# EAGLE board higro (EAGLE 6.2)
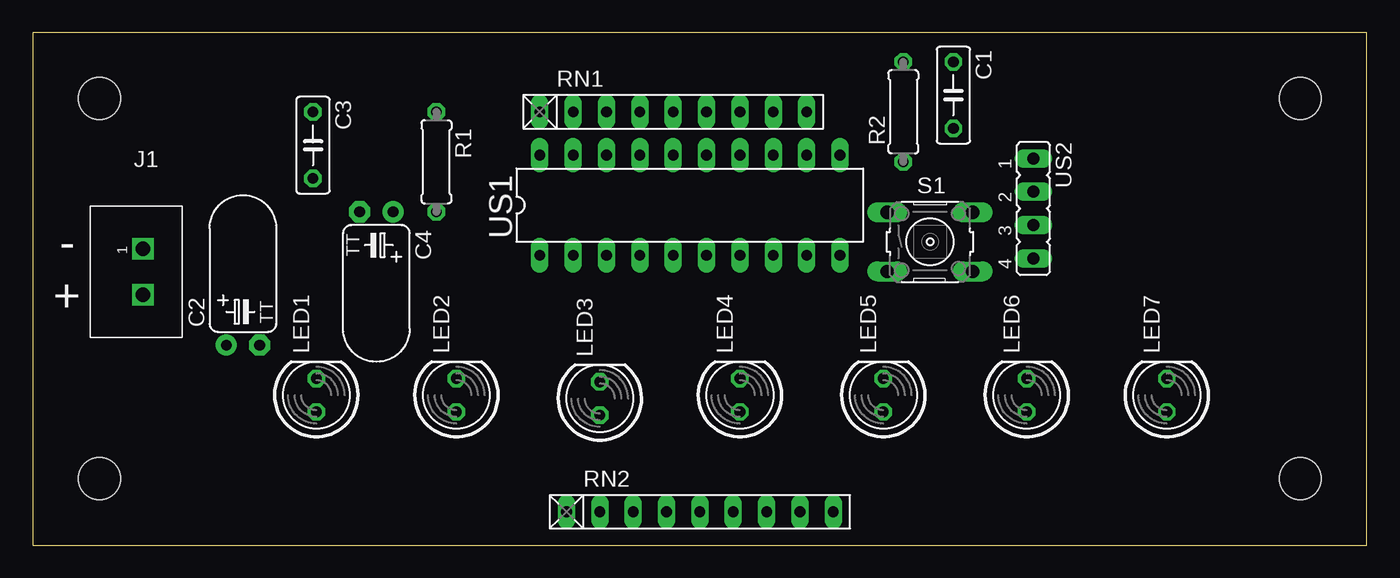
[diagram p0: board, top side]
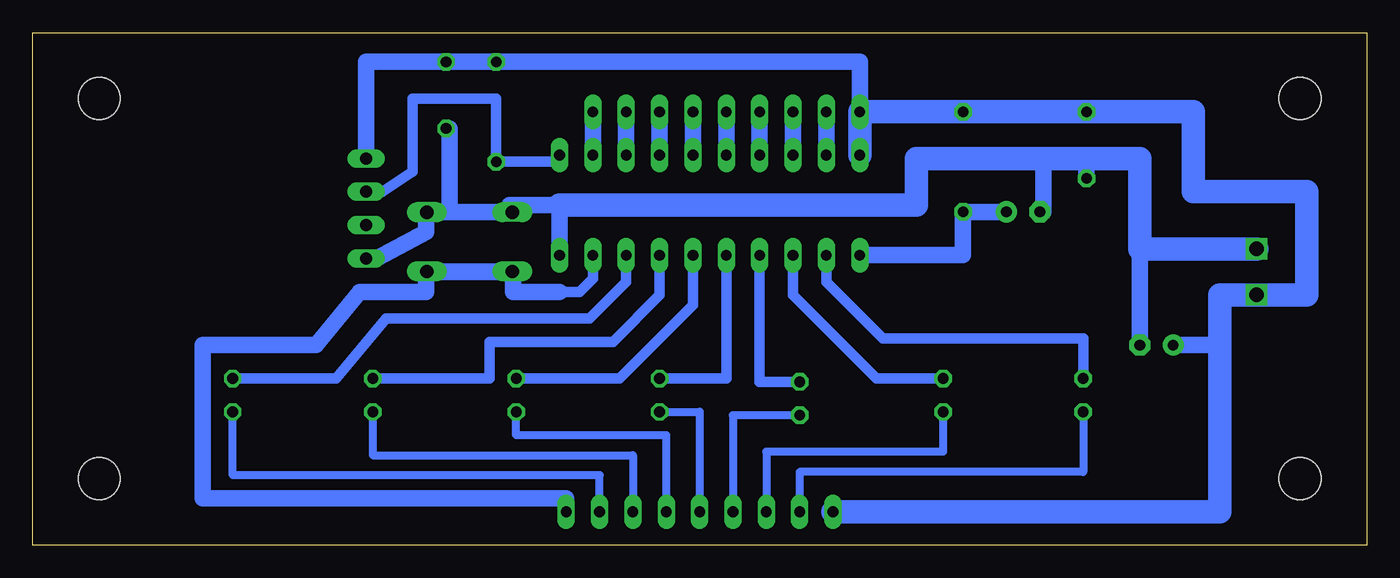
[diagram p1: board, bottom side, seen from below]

Size 101.58 x 39.04 mm. Coordinates in mm from the lower left corner, seen from the top.
Outline: 0,0 101.58,0 101.58,39.04 0,39.04 0,0
Copper layers (1*16): Top 0.035mm / dielectric 1.5mm / Bottom 0.035mm
Design rules: minimum track width 10mil, minimum drill 24mil, track to track 8mil, track to pad 8mil, pad to pad 8mil, via to via 8mil, smd to smd 8mil, copper to edge 40mil, drill to drill 8mil, minimum pad ring 10mil, minimum via ring 8mil, stop-mask expansion 4mil, vias tented up to drill 0mil, thermal gap 10mil
Holes 3.2 mm at 5.08,5.08 96.52,5.08 5.08,34.04 96.52,34.04

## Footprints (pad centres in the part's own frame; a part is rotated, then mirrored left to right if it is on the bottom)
C050-025X075 = drill 0.813 octagon: 1 -2.54,0; 2 2.54,0
TT2D5L = drill 0.813 pad 1.6: + -1.27,0 | drill 0.813 pad 1.6 octagon: - 1.27,0
2PIN-3,5MM = drill 1.1 square: P$1 -1.75,0; P$2 1.75,0
LED5MM = drill 0.813 octagon: A -1.27,0; K 1.27,0
0207/7 = drill 0.813 octagon: 1 -3.81,0; 2 3.81,0
RN-9 = drill 0.813 long: 1 -10.16,0; 2 -7.62,0; 3 -5.08,0; 4 -2.54,0; 5 0,0; 6 2.54,0; 7 5.08,0; 8 7.62,0; 9 10.16,0
B3F-10XX = drill 1.016 long: 1 -3.251,2.261; 2 3.251,2.261; 3 -3.251,-2.261; 4 3.251,-2.261
DIL20 = drill 0.813 long: 1 -11.43,-3.81; 2 -8.89,-3.81; 3 -6.35,-3.81; 4 -3.81,-3.81; 5 -1.27,-3.81; 6 1.27,-3.81; 7 3.81,-3.81; 8 6.35,-3.81; 9 8.89,-3.81; 10 11.43,-3.81; 11 11.43,3.81; 12 8.89,3.81; 13 6.35,3.81; 14 3.81,3.81; 15 1.27,3.81; 16 -1.27,3.81; 17 -3.81,3.81; 18 -6.35,3.81; 19 -8.89,3.81; 20 -11.43,3.81
JP4 = drill 0.914 long: 1 -3.81,0; 2 -1.27,0; 3 1.27,0; 4 3.81,0

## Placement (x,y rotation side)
C1  100n  [C050-025X075]  70.1,34.29 270 top
C2  22u  [TT2D5L]  16,15.24 0 top
C3  100n  [C050-025X075]  21.34,30.48 270 top
C4  22u  [TT2D5L]  26.16,25.4 180 top
J1  ARK2-3,5MM  [2PIN-3,5MM]  8.38,20.83 270 top
LED1  [LED5MM]  21.59,11.43 90 top
LED2  [LED5MM]  32.26,11.43 90 top
LED3  [LED5MM]  43.18,11.18 90 top
LED4  [LED5MM]  53.85,11.43 90 top
LED5  [LED5MM]  64.77,11.43 90 top
LED6  [LED5MM]  75.69,11.43 90 top
LED7  [LED5MM]  86.36,11.43 90 top
R1  3,3k  [0207/7]  30.73,29.21 270 top
R2  3,3k  [0207/7]  66.29,33.02 90 top
RN1  8x470  [RN-9]  48.77,33.02 0 top
RN2  8x470  [RN-9]  50.8,2.54 0 top
S1  [B3F-10XX]  68.33,23.11 0 top
US1  ATTINY2313P  [DIL20]  50.04,25.91 0 top
US2  DHT11  [JP4]  76.2,25.65 270 top

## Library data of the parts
C1-C4 R1 R2 = rcl
J1 = zlacza_futrzak
LED1-LED7 = led
RN1 RN2 = inne_futrzak
S1 = switch-omron; MPN: B3F-1000; OC_FARNELL: 176432; OC_NEWARK: 36M3542
US1 = scalaki_futrzak; OC_FARNELL: unknown; OC_NEWARK: unknown
US2 = jumper

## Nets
+5V: C1.1 C2.+ C3.1 J1.P$2 R1.1 R2.2 RN1.1 RN2.1 US1.20 US2.1
GND: C1.2 C2.- C3.2 C4.- J1.P$1 S1.1 S1.2 US1.10 US2.4
N$1: LED1.K US1.2
N$2: LED2.K US1.3
N$3: LED3.K US1.4
N$4: LED4.K US1.5
N$5: LED5.K US1.6
N$6: LED6.K US1.7
N$7: LED7.K US1.8
N$8: RN1.2 US1.19
N$9: LED7.A RN2.8
N$10: LED6.A RN2.7
N$11: LED5.A RN2.6
N$12: LED4.A RN2.5
N$13: LED3.A RN2.4
N$14: LED2.A RN2.3
N$15: LED1.A RN2.2
N$16: RN1.3 US1.18
N$17: RN1.4 US1.17
N$18: RN1.5 US1.16
N$19: RN1.6 US1.15
N$20: RN1.7 US1.14
N$21: RN1.8 US1.13
N$22: RN1.9 US1.12
N$23: R2.1 US1.11 US2.2
N$24: RN2.9 S1.3 S1.4 US1.9
N$27: C4.+ R1.2 US1.1

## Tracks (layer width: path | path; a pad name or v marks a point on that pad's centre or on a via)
+5V
  Bottom 1.27: RN1.1 38.61,36.83 R2.2 C1.1 76.2,36.83 US2.1 | C2.+ 11.18,15.24 11.18,14.99
  Bottom 1.778: RN2.1 11.18,2.54 11.18,14.99 11.18,19.05 8.38,19.05 | US1.20 RN1.1 R1.1 C3.1 13.21,33.02 13.21,26.92 4.57,26.92 4.57,19.05 8.38,19.05 | 8.38,19.05 J1.P$2
GND
  Bottom 1.27: 69.85,25.38 S1.2 71.63,25.38 71.63,23.88 75.39,21.84 US2.4 | 69.85,25.38 S1.1 65.28,25.88 65.28,25.91 61.47,25.91 US1.10 | C3.2 21.34,29.46 | C4.- 24.64,25.4 24.64,29.46 | 17.27,22.58 C2.- | C1.2 69.85,31.75 69.85,25.38
  Bottom 1.778: 61.47,25.91 34.29,25.91 34.29,29.46 24.64,29.46 21.34,29.46 17.27,29.46 17.27,22.58 J1.P$1
N$1
  Bottom 0.813: US1.2 41.15,20.07 36.83,15.75 21.59,15.75 LED1.K
N$2
  Bottom 0.813: LED2.K 37.34,12.7 43.69,19.05 US1.3
N$3
  Bottom 0.813: LED3.K 46.23,12.45 US1.4
N$4
  Bottom 0.813: LED4.K 48.77,12.7 US1.5
N$5
  Bottom 0.813: LED5.K 56.9,12.7 51.31,18.29 US1.6
N$6
  Bottom 0.813: LED6.K 66.8,12.7 66.8,15.49 57.4,15.49 53.85,19.05 US1.7
N$7
  Bottom 0.813: LED7.K 78.49,12.7 74.68,17.27 59.18,17.27 56.39,20.07 US1.8
N$8
  Bottom 1.27: RN1.2 US1.19
N$9
  Bottom 0.61: RN2.8 58.42,5.33 86.36,5.33 LED7.A
N$10
  Bottom 0.61: LED6.A 75.69,6.86 55.88,6.86 RN2.7
N$11
  Bottom 0.61: RN2.6 53.34,8.38 64.77,8.38 LED5.A
N$12
  Bottom 0.61: LED4.A 50.8,10.16 RN2.5
N$13
  Bottom 0.61: LED3.A 48.26,9.91 RN2.4
N$14
  Bottom 0.61: LED2.A 32.26,7.11 45.72,7.11 RN2.3
N$15
  Bottom 0.61: LED1.A 21.59,5.59 43.18,5.59 RN2.2
N$16
  Bottom 1.27: RN1.3 US1.18
N$17
  Bottom 1.27: RN1.4 US1.17
N$18
  Bottom 1.27: RN1.5 US1.16
N$19
  Bottom 1.27: US1.15 RN1.6
N$20
  Bottom 1.27: US1.14 RN1.7
N$21
  Bottom 1.27: RN1.8 US1.13
N$22
  Bottom 1.27: RN1.9 US1.12
N$23
  Bottom 0.813: US1.11 61.47,29.21 R2.1 66.29,34.04 72.64,34.04 72.64,28.45 74.93,26.92 US2.2
N$24
  Bottom 0.813: 61.47,19.3 59.94,19.3 58.93,20.32 US1.9
  Bottom 1.27: RN2.9 60.96,3.56 88.65,3.56 88.65,15.24 80.01,15.24 76.71,19.3 71.63,19.3 71.63,20.83 65.08,20.83 | 61.47,19.3 65.02,19.3 65.02,20.83 65.08,20.83 | S1.4 S1.3 65.08,20.83
N$27
  Bottom 1.27: US1.1 30.73,22.1 R1.2 C4.+

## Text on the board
tPlace: - | +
